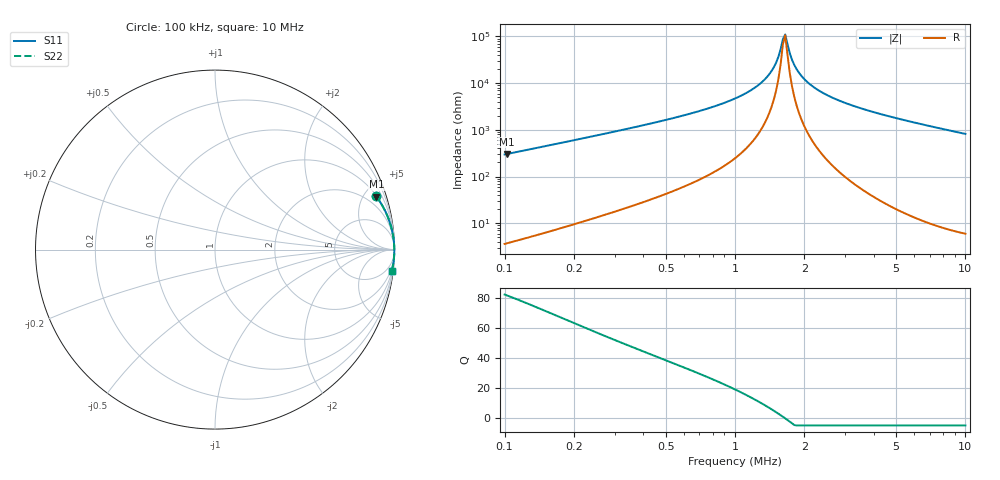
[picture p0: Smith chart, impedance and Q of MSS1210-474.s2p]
# MHz S MA R 50
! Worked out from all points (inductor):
!   203 points, 100 kHz to 10 MHz, reference 50 ohm
!   read as one part in series: L = 470 uH near 102.3 kHz
!   highest Q = 81.7 at 102.3 kHz (marker M1), where L = 472 uH
!   self-resonance near 1.614 MHz
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0.1  0.9441 18.6  0.3185 -70.7  0.3185 -70.7  0.9441 18.6
0.102306  0.9463 18.2  0.312 -71.1  0.312 -71.1  0.9463 18.2
0.2121938  0.9855 8.9  0.1547 -80.2  0.1547 -80.2  0.9855 8.9
0.3751953  0.9945 4.9  0.08513 -83.9  0.08513 -83.9  0.9945 4.9
1.095479  0.9988 1.0  0.01718 -85.4  0.01718 -85.4  0.9988 1.0
1.344971  0.999 0.5  0.008346 -82.9  0.008346 -82.9  0.999 0.5
1.440177  0.999 0.3  0.005511 -79.9  0.005511 -79.9  0.999 0.3
1.507363  0.9991 0.2  0.003657 -75.3  0.003657 -75.3  0.9991 0.2
1.577683  0.9991 0.1  0.001884 -61.5  0.001884 -61.5  0.9991 0.1
1.614064  0.9991 0.0  0.00114 -38.9  0.00114 -38.9  0.9991 0.0
1.651284  0.9991 -0.0  0.0009063 14.3  0.0009063 14.3  0.9991 -0.0
1.728318  0.9991 -0.1  0.002274 67.7  0.002274 67.7  0.9991 -0.1
1.768173  0.9991 -0.2  0.003164 74.2  0.003164 74.2  0.9991 -0.2
1.85066  0.9992 -0.3  0.005006 80.1  0.005006 80.1  0.9992 -0.3
1.936996  0.9992 -0.4  0.006884 82.8  0.006884 82.8  0.9992 -0.4
2.272143  0.9991 -0.8  0.01364 86.0  0.01364 86.0  0.9991 -0.8
2.726739  0.9991 -1.2  0.02182 86.9  0.02182 86.9  0.9991 -1.2
3.424944  0.9988 -1.9  0.03311 87.0  0.03311 87.0  0.9988 -1.9
5.162633  0.9977 -3.3  0.05818 86.0  0.05818 86.0  0.9977 -3.3
6.787083  0.9961 -4.6  0.07998 84.9  0.07998 84.9  0.9961 -4.6
8.524974  0.994 -5.9  0.1025 83.7  0.1025 83.7  0.994 -5.9
10  0.9917 -7.0  0.1213 82.6  0.1213 82.6  0.9917 -7.0
